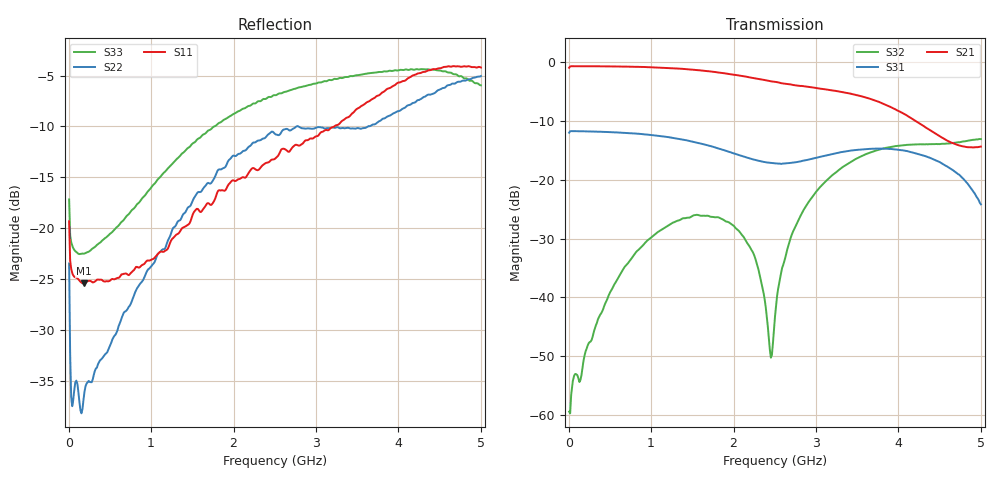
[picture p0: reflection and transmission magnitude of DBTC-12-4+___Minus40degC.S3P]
! Mini-Circuits
! S3P DATA File Format
! Type: Directional Coupler
! Model:DBTC-12-4+
! PINOUT: IN PORT=PORT1 , OUT PORT=PORT2 , COUPLED PORT=PORT3
! TEST CONDITIONS: INPUT POWER = 0 dBm @ Temperature = - 40 deg C
! 401 Frequency points
! All S Parameters are in dB deg format
# MHz S DB R 50
!FREQ	MAG(S11)PHS(S11)MAG(S12)PHS(S12)MAG(S13)PHS(S13)
!	MAG(S21)PHS(S21)MAG(S22)PHS(S22)MAG(S23)PHS(S23)
!	MAG(S31)PHS(S31)MAG(S32)PHS(S32)MAG(S33)PHS(S33)
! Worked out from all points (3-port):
!   401 points, 5 MHz to 5 GHz, reference 50 ohm
!   strongest paths, dB at 5 MHz, 1.254 GHz, 2.502 GHz, 3.751 GHz, 5 GHz:
!     S21: -0.9, -1.0, -3.3, -6.7, -14.3
!     S31: -12.0, -12.8, -17.2, -14.7, -24.1
!     S32: -59.4, -27.3, -43.2, -14.9, -13.1
!   lowest |S11| = -25.4 dB at 179.8 MHz (marker M1), VSWR 1.11, Z = 45.5 + j2.5 ohm
!   |S11| at or under -10 dB: start of sweep to 3.221 GHz
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5  -19.33 148.7  -0.90 3.0  -11.97 -176.5
   -0.92 2.9  -23.47 119.1  -58.92 -179.8
   -11.97 -176.5  -59.43 -172.8  -17.18 150.4
179.83  -25.44 149.2  -0.64 -18.2  -11.75 -205.1
        -0.65 -18.1  -36.85 23.6  -51.60 -462.8
        -11.73 -205.2  -50.74 -456.7  -22.51 167.2
854.15  -23.88 77.4  -0.76 -87.4  -12.18 -298.5
        -0.77 -87.3  -25.60 -90.4  -31.92 -638.3
        -12.16 -298.4  -31.80 -639.0  -17.48 118.6
1540.96  -18.20 15.8  -1.28 -159.6  -13.63 -389.5
         -1.30 -159.4  -16.78 -193.8  -25.97 -747.9
         -13.61 -389.3  -25.97 -748.1  -11.46 37.9
2102.9  -15.02 -52.0  -2.29 -218.8  -15.94 -453.2
        -2.32 -218.5  -12.52 -274.4  -29.38 -836.0
        -15.94 -453.0  -29.40 -836.6  -8.31 -36.1
2502.5  -13.18 -106.4  -3.27 -259.2  -17.13 -486.6
        -3.31 -258.9  -10.74 -327.7  -43.10 -1045.1
        -17.17 -486.5  -43.25 -1042.0  -6.93 -87.5
2714.79  -12.05 -132.9  -3.77 -280.1  -17.02 -502.7
         -3.82 -279.8  -10.26 -358.2  -28.93 -1099.6
         -17.08 -502.5  -29.00 -1099.7  -6.37 -114.5
3189.31  -10.10 -186.5  -4.75 -327.9  -15.62 -547.6
         -4.76 -327.6  -10.12 -421.1  -19.33 -1172.3
         -15.62 -547.7  -19.30 -1172.3  -5.45 -171.1
4163.34  -5.04 -295.2  -9.57 -431.2  -15.33 -673.1
         -9.57 -431.1  -7.75 -546.9  -14.02 -1306.6
         -15.32 -672.7  -13.98 -1306.6  -4.39 -276.5
5000  -4.21 -391.1  -14.22 -471.3  -24.17 -816.9
      -14.33 -471.1  -5.05 -661.5  -13.14 -1399.9
      -24.15 -815.5  -13.06 -1400.2  -5.96 -351.4
